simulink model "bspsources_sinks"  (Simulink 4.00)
settings: Solver=ode45  StartTime=0.0  StopTime=1000.0  FixedStep=0.1  MaxStep=2.0  RelTol=1e-3
libraries: simulink3 x2

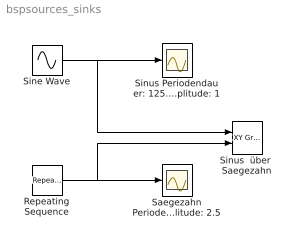
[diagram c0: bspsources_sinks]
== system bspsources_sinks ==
  Repeating Sequence : simulink3/Sources/Repeating Sequence  rep_seq_t=[0 20 40 60 80 100 120 140 160 180 200]  rep_seq_y="[0  0.25 0.5 0.75 1.0 1.25 1.5 1.75 2.0 2.25 2.5 ]"
  Saegezahn Periodendauer: 200s Amplitude: 2.5 : Scope
  Sine Wave : Sin  Amplitude=1  Frequency=0.05  Phase=0  SampleTime=0
  Sinus Periodendauer: 125.664s Amplitude: 1 : Scope
  Sinus  über  Saegezahn : simulink3/Sinks/XY Graph  xmin=-1  xmax=1  ymin=0  ymax=2.5  st=-1
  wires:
  Repeating Sequence/1 -> Saegezahn Periodendauer: 200s Amplitude: 2.5/1, Sinus  über  Saegezahn/2
  Sine Wave/1 -> Sinus  über  Saegezahn/1, Sinus Periodendauer: 125.664s Amplitude: 1/1
